FUNCTION_BLOCK FB_DirectControl EXTENDS FB_AsyncServiceResultClass IMPLEMENTS I_AcsiDataAccessEventClass, I_AcsiDataAccessCompletionClass
VAR
	(* Interface pointer to controllable DO *)
	_ipCtrl					: I_AcsiCommonControllableDataClass;
	(* CDC type of the controllable DO *)
	_eType					: E_AcsiCDCType;
	(* Interface pointer to value of 'Beh' DO of parent LN *)
	_ipBehVal				: I_AcsiDATypeBeh;
	(* Interface pointer to DO containing stepsize information for BAC *)
	_ipStepSize		: I_AcsiDATypeAnalogueValue;
	
	(* State of control state machine *)
	_eControlState			: E_DirectControlState;
	(* Interface pointer to association for the current control procedure *)
	_ipCurrentAA			: I_ScsmAssociationClass;
	(* IP address of the client for the current control procedure *)
	_stCurrrentIp			: ST_SockAddr;
	
	(* Interface pointer to LastApplError request service *)
	_ipLastApplErrorReq		: I_AsyncServiceResultClass;
	(* State of LastApplError transmission *)
	_nLastApplErrorReqState	: BYTE;
	(* Interface pointer to CommandTermination request service *)
	_ipCmdTermReq			: I_AsyncServiceResultClass;
	(* State of CommandTermination transmission *)
	_nCmdTermReqState		: BYTE;
	
	(* Indicates whether this function block has been initialized *)
	bInit					: BOOL;
	(* Indicates whether the ControlState changed in the last cycle *)
	bNewState				: BOOL;
	(* Indicates whether a valid Oper_req was received *)
	bOperReq				: BOOL;
	(* Token for CompletionWaitEvent *)
	fbCompletion			: FB_AcsiServiceResultClass;
END_VAR

(*
	Checks if the value of 'Oper.ctlVal' is valid.
	Return value: TRUE => success, FALSE => failure
*)
METHOD PROTECTED _CheckCtlVal : BOOL
VAR_INPUT
	(* Value of 'ctlVal' DA *)
	uCtlVal			: U_AcsiCtlVal;
END_VAR
VAR_OUTPUT
	(* Error *)
	eError			: E_AcsiApplError;
	(* Application error code *)
	eAddCause		: E_AcsiApplAddCause;
END_VAR
IF (_ipCtrl = 0) OR_ELSE (_eType = E_AcsiCDCType.none) THEN
	RETURN;
END_IF

CASE _eType OF
	E_AcsiCDCType.SPC:
		IF (_ipCtrl.ipStVal_BOOLEAN = 0) THEN
			RETURN;
		END_IF
		IF (uCtlVal.SPC = _ipCtrl.ipStVal_BOOLEAN.bValue) THEN
			eError:=E_AcsiApplError.NoError;
			eAddCause:=E_AcsiApplAddCause.PositionReached;
		ELSE
			_CheckCtlVal:=TRUE;
		END_IF
	
	E_AcsiCDCType.DPC:
		IF (_ipCtrl.ipStVal_Dbpos = 0) THEN
			RETURN;
		END_IF
		IF ((SEL(uCtlVal.DPC, E_AcsiDbpos.Off, E_AcsiDbpos.On)) = _ipCtrl.ipStVal_Dbpos.eValue) THEN
			eError:=E_AcsiApplError.NoError;
			eAddCause:=E_AcsiApplAddCause.PositionReached;
		ELSE
			_CheckCtlVal:=TRUE;
		END_IF
	
	E_AcsiCDCType.INC:
		IF (_ipCtrl.ipStVal_INT32 = 0) THEN
			RETURN;
		END_IF
		IF (uCtlVal.INC = _ipCtrl.ipStVal_INT32.iValue) THEN
			eError:=E_AcsiApplError.NoError;
			eAddCause:=E_AcsiApplAddCause.PositionReached;
		ELSE
			_CheckCtlVal:=TRUE;
		END_IF
		
	E_AcsiCDCType.ENC:
		IF (_ipCtrl.ipStVal_ENUMERATED = 0) THEN
			RETURN;
		END_IF
		IF (uCtlVal.ENC.iAny = _ipCtrl.ipStVal_ENUMERATED.iAny) THEN
			eError:=E_AcsiApplError.NoError;
			eAddCause:=E_AcsiApplAddCause.PositionReached;
		ELSE
			_CheckCtlVal:=TRUE;
		END_IF
	
	E_AcsiCDCType.BSC:
		IF (_ipCtrl.ipValWTr = 0) THEN
			RETURN;
		END_IF
		CASE uCtlVal.BSC OF
			E_AcsiTcmd.Reserved:
				eError:=E_AcsiApplError.NoError;
				eAddCause:=E_AcsiApplAddCause.NotSupported;
			
			E_AcsiTcmd.Lower:
				IF (_ipCtrl.ipValWTr.iPosVal = -64) THEN
					eError:=E_AcsiApplError.NoError;
					eAddCause:=E_AcsiApplAddCause.StepLimit;
				ELSE
					_CheckCtlVal:=TRUE;
				END_IF
			
			E_AcsiTcmd.Higher:
				IF (_ipCtrl.ipValWTr.iPosVal = 63) THEN
					eError:=E_AcsiApplError.NoError;
					eAddCause:=E_AcsiApplAddCause.StepLimit;
				ELSE
					_CheckCtlVal:=TRUE;
				END_IF
			
			E_AcsiTcmd.Stop:
				_CheckCtlVal:=TRUE;
		END_CASE
	
	E_AcsiCDCType.ISC:
		IF (_ipCtrl.ipValWTr = 0) THEN
			RETURN;
		END_IF
		IF (uCtlVal.ISC < -64) OR_ELSE (uCtlVal.ISC > 63) THEN
			eError:=E_AcsiApplError.NoError;
			eAddCause:=E_AcsiApplAddCause.InconsistentParameters;
		ELSE
			_CheckCtlVal:=TRUE;
		END_IF
	
	E_AcsiCDCType.APC:
		IF (_ipCtrl.ipMxVal = 0) THEN
			RETURN;
		ELSE
			_CheckCtlVal:=TRUE;
		END_IF
	
	E_AcsiCDCType.BAC:
		IF (_ipCtrl.ipMxVal = 0) THEN
			RETURN;
		ELSE
			CASE uCtlVal.BAC OF
				E_AcsiTcmd.Reserved:
					eError:=E_AcsiApplError.NoError;
					eAddCause:=E_AcsiApplAddCause.NotSupported;
				
				ELSE
					_CheckCtlVal:=TRUE;
			END_CASE
		END_IF
END_CASE
END_METHOD

(*
	This method performs the operative test.
	Since this test can take multiple PLC cycles, this method is called every cycle, until it returns TRUE.
*)
METHOD PROTECTED _DynamicTest : BOOL
VAR_OUTPUT
	(* Indicates whether the dynamic test was successful *)
	bDynamicTestOk	: BOOL;
	(* Error code for negative response *)
	eError			: E_AcsiServiceError;
END_VAR
bDynamicTestOk:=TRUE;
_DynamicTest:=TRUE;
END_METHOD

(* Initializes necessary local values *)
METHOD PROTECTED _Init
IF (_ipCtrl <> 0) THEN
	(* Set '_eType' according to CDC of the controllable data object *)
	IF (_ipCtrl.sClass = 'SPC') THEN
		_eType:=E_AcsiCDCType.SPC;
	ELSIF (_ipCtrl.sClass = 'DPC') THEN
		_eType:=E_AcsiCDCType.DPC;
	ELSIF (_ipCtrl.sClass = 'INC') THEN
		_eType:=E_AcsiCDCType.INC;
	ELSIF (_ipCtrl.sClass = 'ENC') THEN
		_eType:=E_AcsiCDCType.ENC;
	ELSIF (_ipCtrl.sClass = 'BSC') THEN
		_eType:=E_AcsiCDCType.BSC;
	ELSIF (_ipCtrl.sClass = 'ISC') THEN
		_eType:=E_AcsiCDCType.ISC;
	ELSIF (_ipCtrl.sClass = 'APC') THEN
		_eType:=E_AcsiCDCType.APC;
	ELSIF (_ipCtrl.sClass = 'BAC') THEN
		_eType:=E_AcsiCDCType.BAC;
	END_IF
END_IF
END_METHOD

(*
	This method performs the operative test.
	Since this test can take multiple PLC cycles, this method is called every cycle, until it returns TRUE.
*)
METHOD PROTECTED _OperativeTest : BOOL
VAR_OUTPUT
	(* Indicates whether the operative test was successful *)
	bOperativeTestOk	: BOOL;
	(* Error code for negative response *)
	eError				: E_AcsiServiceError;
END_VAR
VAR
	eApplError			: E_AcsiApplError;
	eApplAddCause		: E_AcsiApplAddCause;
END_VAR
IF (_ipCtrl <> 0) AND_THEN (_ipCtrl.ipOper <> 0) THEN
	(* Don't allow Oper_req if 'ctlModel' is set to 'status-only' *)
	IF (_ipCtrl.ipCtlModel <> 0) AND_THEN (_ipCtrl.ipCtlModel.eValue = E_AcsiCtlModels.StatusOnly) THEN
		_SendLastApplError(ipAA:=_ipCurrentAA,
			ipCtrlData:=_ipCtrl.ipOper,
			eError:=E_AcsiApplError.NoError,
			ipOrigin:=_ipCtrl.ipOper.ipOrigin,
			ipCtlNum:=_ipCtrl.ipOper.ipCtlNum,
			eAddCause:=E_AcsiApplAddCause.Unknown);
		eError:=E_AcsiServiceError.AccessViolation;
	
	(* Check if Oper_req is valid for current value of 'Beh' *)
	ELSIF (_ipBehVal <> 0) AND_THEN ((_ipBehVal.eValue = E_AcsiBeh.Off)
	OR_ELSE ((_ipCtrl.ipOper.ipTest <> 0) AND_THEN (_ipCtrl.ipOper.ipTest.bValue <> ((_ipBehVal.eValue = E_AcsiBeh.Test) OR_ELSE (_ipBehVal.eValue = E_AcsiBeh.TestBlocked))))) THEN
		_SendLastApplError(ipAA:=_ipCurrentAA,
			ipCtrlData:=_ipCtrl.ipOper,
			eError:=E_AcsiApplError.NoError,
			ipOrigin:=_ipCtrl.ipOper.ipOrigin,
			ipCtlNum:=_ipCtrl.ipOper.ipCtlNum,
			eAddCause:=E_AcsiApplAddCause.BlockedByMode);
		eError:=E_AcsiServiceError.AccessViolation;
	
	(* Check if 'ctlVal' is valid *)
	ELSIF (NOT _CheckCtlVal(uCtlVal:=_ipCtrl.ipOper.uCtlVal, eError=>eApplError, eAddCause=>eApplAddCause)) THEN
		_SendLastApplError(ipAA:=_ipCurrentAA,
			ipCtrlData:=_ipCtrl.ipOper,
			eError:=eApplError,
			ipOrigin:=_ipCtrl.ipOper.ipOrigin,
			ipCtlNum:=_ipCtrl.ipOper.ipCtlNum,
			eAddCause:=eApplAddCause);
		eError:=E_AcsiServiceError.AccessViolation;
	
	(* Oper_req is valid *)
	ELSE
		RemoteAddress_From_ScsmAssociation(in:=_ipCurrentAA, out=>_stCurrrentIp);
		bOperativeTestOk:=TRUE;
	END_IF
END_IF
_OperativeTest:=TRUE;
END_METHOD

(* Resets all local values and the ControlState *)
METHOD PROTECTED _Reset
(* Reset local values *)
_ipCurrentAA:=0;
_stCurrrentIp.sAddr:='';
_stCurrrentIp.nPort:=0;
END_METHOD

(* Resets all values of the 'Oper' DA to their configured initial values. *)
METHOD PROTECTED _ResetOperValues
VAR
	(* Interface pointer to 'Oper' DA *)
	ipOper			: I_AcsiDATypeOper;
END_VAR
IF (_ipCtrl = 0) OR_ELSE ((ipOper:=_ipCtrl.ipOper) = 0) THEN
	RETURN;
END_IF

IF (ipOper.ipCtlVal <> 0) THEN
	ipOper.uCtlVal:=ipOper.uCtlVal_Config;
END_IF
IF (ipOper.ipOperTm <> 0) THEN
	ipOper.ipOperTm.tValue:=ipOper.ipOperTm.tConfig;
END_IF
IF (ipOper.ipOrigin <> 0) THEN
	ipOper.ipOrigin.stOrigin:=ipOper.ipOrigin.stConfig;
END_IF
IF (ipOper.ipCtlNum <> 0) THEN
	ipOper.ipCtlNum.nValue:=ipOper.ipCtlNum.nConfig;
END_IF
IF (ipOper.ipT <> 0) THEN
	ipOper.ipT.tValue:=ipOper.ipT.tConfig;
END_IF
IF (ipOper.ipTest <> 0) THEN
	ipOper.ipTest.bValue:=ipOper.ipTest.bConfig;
END_IF
IF (ipOper.ipCheck <> 0) THEN
	ipOper.ipCheck.eValue:=ipOper.ipCheck.eConfig;
END_IF
END_METHOD

(* Sends a negative CommandTermination request *)
METHOD PROTECTED _SendCommandTerminationReqNeg : BOOL
VAR_INPUT
	(* Interface pointer to application association *)
	ipAA			: I_ScsmAssociationClass;
	(* Interface pointer to 'Oper', 'Cancel' or 'SBOw' control object, e.g. 'Relay1/XCBR1.CO.Pos.Oper', 'Relay1/CSWI1.CO.Pos.Cancel', 'Relay1/XCBR1.CO.Pos.SBOw' *)
	ipCtrlData		: I_AcsiCommonDataClass;
	(* Error *)
	eError			: E_AcsiApplError;
	(* Interface pointer to 'origin' attribute *)
	ipOrigin		: I_AcsiDATypeOriginator;
	(* Interface pointer to 'ctlNum' attribute *)
	ipCtlNum		: I_AcsiBAtypeINT8U;
	(* Application error code *)
	eAddCause		: E_AcsiApplAddCause;
END_VAR
VAR
	ipLastApplError	:I_AcsiDATypeLastApplError;
END_VAR
IF (ipAA <> 0)
AND_THEN (ipCtrlData <> 0)
AND_THEN (ipOrigin <> 0)
AND_THEN (ipCtlNum <> 0) THEN
	ipLastApplError:=ipAA.SetAdditionalCauseDiag(ipCtrlData:=ipCtrl,
		eError:=eError,
		stOrigin:=ipOrigin.stOrigin,
		nCtlNum:=ipCtlNum.nValue,
		eAddCause:=eAddCause);
	ipAA.CommandTerminationReq(ipCtrlData:=ipCtrlData,
		ipLastApplError:=ipLastApplError,
		ipResult=>_ipCmdTermReq);
	_nCmdTermReqState:=1;
END_IF
END_METHOD

(* Sends a positive CommandTermination request *)
METHOD PROTECTED _SendCommandTerminationReqPos : BOOL
VAR_INPUT
	(* Interface pointer to application association *)
	ipAA			: I_ScsmAssociationClass;
	(* Interface pointer to 'Oper', 'Cancel' or 'SBOw' control object, e.g. 'Relay1/XCBR1.CO.Pos.Oper', 'Relay1/CSWI1.CO.Pos.Cancel', 'Relay1/XCBR1.CO.Pos.SBOw' *)
	ipCtrlData		: I_AcsiCommonDataClass;
END_VAR
IF (ipAA <> 0)
AND_THEN (ipCtrlData <> 0) THEN
	_SendCommandTerminationReqPos:=ipAA.CommandTerminationReq(ipCtrlData:=ipCtrlData,
		ipLastApplError:=0,
		ipResult=>_ipCmdTermReq);
	_nCmdTermReqState:=1;
END_IF
END_METHOD

(* Sends a LastApplError request *)
METHOD PROTECTED _SendLastApplError : BOOL
VAR_INPUT
	(* Interface pointer to application association *)
	ipAA			: I_ScsmAssociationClass;
	(* Interface pointer to 'Oper', 'Cancel' or 'SBOw' control object *)
	ipCtrlData		: I_AcsiCommonDataClass;
	(* Error *)
	eError			: E_AcsiApplError;
	(* Interface pointer to 'origin' attribute *)
	ipOrigin		: I_AcsiDATypeOriginator;
	(* Interface pointer to 'ctlNum' attribute *)
	ipCtlNum		: I_AcsiBAtypeINT8U;
	(* Application error code *)
	eAddCause		: E_AcsiApplAddCause;
END_VAR
VAR
	(* Interface pointer to AdditionalCauseDiag object *)
	ipLastApplError	: I_AcsiDATypeLastApplError;
END_VAR
(* Get values from 'Oper' and send LastApplError *)
IF (ipAA <> 0) AND_THEN (ipOrigin <> 0) AND_THEN (ipCtlNum <> 0) THEN
	ipLastApplError:=ipAA.SetAdditionalCauseDiag(ipCtrlData:=ipCtrlData,
		eError:=eError,
		stOrigin:=ipOrigin.stOrigin,
		nCtlNum:=ipCtlNum.nValue,
		eAddCause:=eAddCause);
		
	_SendLastApplError:=ipAA.LastApplErrorReq(ipLastApplError:=ipLastApplError, ipResult=>_ipLastApplErrorReq);
	SUPER^.SetBusy();
	_nLastApplErrorReqState:=1;
END_IF
END_METHOD

(*
	Sets the value of 'mxVal' to the value of 'ctlVal'.
	Return value: TRUE => success, FALSE => failure
*)
METHOD PROTECTED _SetApcValue : BOOL
VAR_INPUT
	(* Interface pointer to DA that will be written *)
	ipMxVal			: I_AcsiDATypeAnalogueValue;
	(* Value of 'ctlVal' DA *)
	uCtlVal			: U_AcsiCtlVal;
	(* Interface pointer to 'ctlVal' of type AnalogueValue *)
	ipCtlVal_AV		: I_AcsiDATypeAnalogueValue;
END_VAR
VAR
END_VAR
IF ((ipMxVal = 0) OR_ELSE ((ipMxVal.ipF = 0) AND_THEN (ipMxVal.ipI = 0)))
OR_ELSE ((ipCtlVal_AV = 0) OR_ELSE ((ipCtlVal_AV.ipF = 0) AND_THEN (ipCtlVal_AV.ipI = 0))) THEN
	RETURN;
END_IF

IF (ipMxVal.ipF <> 0) THEN
	IF (ipCtlVal_AV.ipF <> 0) THEN
		ipMxVal.fValue:=uCtlVal.APC.f;
	ELSE
		(* 'ctlVal.i' is present, but not 'ctlVal.f' -> convert and use value of 'ctlVal.i' *)
		ipMxVal.fValue:=DINT_TO_REAL(uCtlVal.APC.i);
	END_IF
END_IF
IF (ipMxVal.ipI <> 0) THEN
	IF (ipCtlVal_AV.ipI <> 0) THEN
		ipMxVal.iValue:=uCtlVal.APC.i;
	ELSE
		(* 'ctlVal.f' is present, but not 'ctlVal.i' -> convert and use value of 'ctlVal.f' *)
		ipMxVal.iValue:=REAL_TO_DINT(uCtlVal.APC.f);
	END_IF
END_IF
_SetApcValue:=TRUE;
END_METHOD

(*
	Increments or decrements the value of 'mxVal' according to the value of 'ctlVal' and 'stepSize'.
	If 'stepSize' is not specified, the value 1 is used.
	Return value: TRUE => success, FALSE => failure
*)
METHOD PROTECTED _SetBacValue : BOOL
VAR_INPUT
	(* Interface pointer to DA that will be written *)
	ipMxVal			: I_AcsiDATypeAnalogueValue;
	(* Value of 'ctlVal' DA *)
	uCtlVal			: U_AcsiCtlVal;
	(* Interface pointer to 'stepSize' DA (Optional) *)
	ipStepSize		: I_AcsiDATypeAnalogueValue;
END_VAR
VAR
	(* stepSize for 'f' *)
	fStepSize		: REAL:=1.0;
	(* stepSize for 'i' *)
	iStepSize		: DINT:=1;
END_VAR
IF (ipMxVal = 0) OR_ELSE ((ipMxVal.ipF = 0) AND_THEN (ipMxVal.ipI = 0)) THEN
	RETURN;
END_IF

IF (ipStepSize <> 0) AND_THEN (((ipStepSize.ipF <> 0) AND_THEN (ipStepSize.fValue <> 0.0)) OR_ELSE ((ipStepSize.ipI <> 0) AND_THEN (ipStepSize.iValue <> 0))) THEN
	IF (ipStepSize.ipF <> 0) THEN
		fStepSize:=ipStepSize.fValue;
	ELSE
		(* 'stepSize.i' is present, but not 'stepSize.f' -> convert and use value of 'stepSize.i' *)
		fStepSize:=DINT_TO_REAL(ipStepSize.iValue);
	END_IF
	IF (ipStepSize.ipI <> 0) THEN
		iStepSize:=ipStepSize.iValue;
	ELSE
		(* 'stepSize.f' is present, but not 'stepSize.i' -> convert and use value of 'stepSize.f' *)
		iStepSize:=REAL_TO_DINT(ipStepSize.fValue);
	END_IF
END_IF

CASE uCtlVal.BAC OF
	E_AcsiTcmd.Stop:
		_SetBacValue:=TRUE;
	
	E_AcsiTcmd.Lower:
		IF (ipMxVal.ipF <> 0) THEN
			ipMxVal.fValue:=ipMxVal.fValue - fStepSize;
		END_IF
		IF (ipMxVal.ipI <> 0) THEN
			ipMxVal.iValue:=ipMxVal.iValue - iStepSize;
		END_IF
		_SetBacValue:=TRUE;
	
	E_AcsiTcmd.Higher:
		IF (ipMxVal.ipF <> 0) THEN
			ipMxVal.fValue:=ipMxVal.fValue + fStepSize;
		END_IF
		IF (ipMxVal.ipI <> 0) THEN
			ipMxVal.iValue:=ipMxVal.iValue + iStepSize;
		END_IF
		_SetBacValue:=TRUE;
END_CASE
END_METHOD

(*
	Increments or decrements the value of 'valWTr' according to the value of 'ctlVal'.
	Return value: TRUE => success, FALSE => failure
*)
METHOD PROTECTED _SetBscValue : BOOL
VAR_INPUT
	(* Interface pointer to DA that will be written *)
	ipValWTr		: I_AcsiDATypeValWithTrans;
	(* Value of 'ctlVal' DA *)
	uCtlVal			: U_AcsiCtlVal;
END_VAR
VAR
END_VAR
IF (ipValWTr = 0) THEN
	RETURN;
END_IF

CASE uCtlVal.BSC OF
	E_AcsiTcmd.Stop:
		_SetBscValue:=TRUE;
	
	E_AcsiTcmd.Lower:
		ipValWTr.iPosVal:=ipValWTr.iPosVal - 1;
		_SetBscValue:=TRUE;
	
	E_AcsiTcmd.Higher:
		ipValWTr.iPosVal:=ipValWTr.iPosVal + 1;
		_SetBscValue:=TRUE;
END_CASE
END_METHOD

(*
	Sets the value of 'stVal' according to the value of 'ctlVal'.
	Return value: TRUE => success, FALSE => failure
*)
METHOD PROTECTED _SetDpcValue : BOOL
VAR_INPUT
	(* Interface pointer to DA that will be written *)
	ipStVal			: I_AcsiDATypeDbpos;
	(* Value of 'ctlVal' DA *)
	uCtlVal			: U_AcsiCtlVal;
END_VAR
VAR
END_VAR
IF (ipStVal = 0) THEN
	RETURN;
END_IF

ipStVal.eValue:=SEL(uCtlVal.DPC, E_AcsiDbpos.Off, E_AcsiDbpos.On);
_SetDpcValue:=TRUE;
END_METHOD

(*
	Sets the value of 'stVal' to the value of 'ctlVal'.
	Return value: TRUE => success, FALSE => failure
*)
METHOD PROTECTED _SetEncValue : BOOL
VAR_INPUT
	(* Interface pointer to DA that will be written *)
	ipStVal			: I_AcsiBATypeENUMERATED;
	(* Value of 'ctlVal' DA *)
	uCtlVal			: U_AcsiCtlVal;
END_VAR
VAR
END_VAR
IF (ipStVal = 0) THEN
	RETURN;
END_IF

ipStVal.iAny:=uCtlVal.ENC.iAny;
_SetEncValue:=TRUE;
END_METHOD

(*
	Sets the value of 'stVal' to the value of 'ctlVal'.
	Return value: TRUE => success, FALSE => failure
*)
METHOD PROTECTED _SetIncValue : BOOL
VAR_INPUT
	(* Interface pointer to DA that will be written *)
	ipStVal			: I_AcsiBATypeINT32;
	(* Value of 'ctlVal' DA *)
	uCtlVal			: U_AcsiCtlVal;
END_VAR
VAR
END_VAR
IF (ipStVal = 0) THEN
	RETURN;
END_IF

ipStVal.iValue:=uCtlVal.INC;
_SetIncValue:=TRUE;
END_METHOD

(*
	Sets the value of 'valWTr' to the value of 'ctlVal'.
	Return value: TRUE => success, FALSE => failure
*)
METHOD PROTECTED _SetIscValue : BOOL
VAR_INPUT
	(* Interface pointer to DA that will be written *)
	ipValWTr		: I_AcsiDATypeValWithTrans;
	(* Value of 'ctlVal' DA *)
	uCtlVal			: U_AcsiCtlVal;
END_VAR
VAR
END_VAR
IF (ipValWTr = 0) THEN
	RETURN;
END_IF

ipValWTr.iPosVal:=uCtlVal.ISC;
_SetIscValue:=TRUE;
END_METHOD

(*
	Sets the value of 'stVal' to the value of 'ctlVal'.
	Return value: TRUE => success, FALSE => failure
*)
METHOD PROTECTED _SetSpcValue : BOOL
VAR_INPUT
	(* Interface pointer to DA that will be written *)
	ipStVal			: I_AcsiBATypeBOOLEAN;
	(* Value of 'ctlVal' DA *)
	uCtlVal			: U_AcsiCtlVal;
END_VAR
VAR
END_VAR
IF (ipStVal = 0) THEN
	RETURN;
END_IF

ipStVal.bValue:=uCtlVal.SPC;
_SetSpcValue:=TRUE;
END_METHOD

(*
	Sets the value of the respective DA according to the value of 'Oper.ctlVal'.
	Return value: TRUE => success, FALSE => failure
*)
METHOD PROTECTED _SetValue : BOOL
VAR_INPUT
	(* Value of 'ctlVal' DA *)
	uCtlVal			: U_AcsiCtlVal;
	(* Interface pointer to 'ctlVal' of type AnalogueValue *)
	ipCtlVal_AV		: I_AcsiDATypeAnalogueValue;
END_VAR
IF (_ipCtrl = 0) THEN
	RETURN;
END_IF

CASE _eType OF
	E_AcsiCDCType.SPC:
		_SetValue:=_SetSpcValue(ipStVal:=_ipCtrl.ipStVal_BOOLEAN, uCtlVal:=uCtlVal);
	
	E_AcsiCDCType.DPC:
		_SetValue:=_SetDpcValue(ipStVal:=_ipCtrl.ipStVal_Dbpos, uCtlVal:=uCtlVal);
	
	E_AcsiCDCType.INC:
		_SetValue:=_SetIncValue(ipStVal:=_ipCtrl.ipStVal_INT32, uCtlVal:=uCtlVal);
	
	E_AcsiCDCType.ENC:
		_SetValue:=_SetEncValue(ipStVal:=_ipCtrl.ipStVal_ENUMERATED, uCtlVal:=uCtlVal);
	
	E_AcsiCDCType.BSC:
		_SetValue:=_SetBscValue(ipValWTr:=_ipCtrl.ipValWTr, uCtlVal:=uCtlVal);
	
	E_AcsiCDCType.ISC:
		_SetValue:=_SetIscValue(ipValWTr:=_ipCtrl.ipValWTr, uCtlVal:=uCtlVal);
	
	E_AcsiCDCType.APC:
		_SetValue:=_SetApcValue(ipMxVal:=_ipCtrl.ipMxVal, uCtlVal:=uCtlVal, ipCtlVal_AV:=ipCtlVal_AV);
	
	E_AcsiCDCType.BAC:
		_SetValue:=_SetBacValue(ipMxVal:=_ipCtrl.ipMxVal, uCtlVal:=uCtlVal, ipStepSize:=_ipStepSize);
END_CASE
END_METHOD

(*
	Sets the value of 't' to the current time.
	Return value: TRUE => success, FALSE => failure
*)
METHOD PROTECTED _UpdateTimestampValue : BOOL
VAR_INPUT
	(* Interface pointer to association *)
	ipAA			: I_ScsmAssociationClass;
END_VAR
VAR
	(* Current time *)
	tValue			: T_UtcTime;
END_VAR
IF (ipAA <> 0) AND_THEN (_ipCtrl <> 0) AND_THEN (_ipCtrl.ipT <> 0) THEN
	_UpdateTimestampValue:=ipAA.GetSystemTime(tT=>tValue);
	_ipCtrl.ipT.tValue:=tValue;
END_IF
END_METHOD

PROPERTY eType : E_AcsiCDCType
GET
eType:=_eType;
END_GET
SET
_eType:=eType;
END_SET
END_PROPERTY

METHOD Execute : BOOL
VAR
	(* Used to cache the return value of the last '_OperativeTest' or '_DynamicTest' method call *)
	bTestOk	: BOOL;
	(* Used to cache the returned error of the last '_OperativeTest' or '_DynamicTest' method call *)
	eError	: E_AcsiServiceError;
	
	(* Used to cache the current system time for 'tOpOk' *)
	tValue	: T_UtcTime;
END_VAR
IF (_ipCtrl <> 0) AND_THEN (_ipCtrl.ipOper <> 0) THEN
	(* Initialize function block in the first cycle *)
	IF NOT bInit THEN
		_Init();
		bInit:=TRUE;
	END_IF
	
	CASE _eControlState OF
		E_DirectControlState.Ready:
			(* Check if ControlState changed in the last cycle *)
			IF bNewState THEN
				bNewState:=FALSE;
				_Reset();
			END_IF
			(* Check if a valid Oper_req was received *)
			IF bOperReq THEN
				bOperReq:=FALSE;
				(* Go to next ControlState *)
				_eControlState:=E_DirectControlState.PerformTest;
				bNewState:=TRUE;
			END_IF
		
		E_DirectControlState.PerformTest:
			(* Check if ControlState changed in the last cycle *)
			IF bNewState THEN
				bNewState:=FALSE;
				(* Set 'opRcvd' *)
				IF (_ipCtrl.ipOpRcvd <> 0) THEN
					_ipCtrl.ipOpRcvd.bValue:=TRUE;
				END_IF
			END_IF
			(* Trigger the operative test until it is finished *)
			IF _OperativeTest(bOperativeTestOk=>bTestOk, eError=>eError) THEN
				(* Reset 'opRcvd' *)
				IF (_ipCtrl.ipOpRcvd <> 0) THEN
					_ipCtrl.ipOpRcvd.bValue:=FALSE;
				END_IF
				IF bTestOk THEN
					(* Go to next ControlState *)
					_eControlState:=E_DirectControlState.WaitForExecution;
				ELSE
					fbCompletion.SetCompleted();
					fbCompletion.eServiceError:=eError;
					(* Go back to ControlState 'Ready' *)
					_eControlState:=E_DirectControlState.Ready;
				END_IF
				bNewState:=TRUE;
			END_IF
		
		E_DirectControlState.WaitForExecution:
			(* Check if ControlState changed in the last cycle *)
			IF bNewState THEN
				bNewState:=FALSE;
			END_IF
			(* Trigger the dynamic test until it is finished *)
			IF _DynamicTest(bDynamicTestOk=>bTestOk, eError=>eError) THEN
				fbCompletion.SetCompleted();
				IF bTestOk THEN
					(* Go to next ControlState *)
					IF (_ipBehVal <> 0) AND_THEN ((_ipBehVal.eValue = E_AcsiBeh.TestBlocked) OR_ELSE (_ipBehVal.eValue = E_AcsiBeh.OnBlocked)) THEN
						_eControlState:=E_DirectControlState.MirrorBlockedCommand;
					ELSE
						_eControlState:=E_DirectControlState.WaitForChange;
					END_IF
				ELSE
					fbCompletion.eServiceError:=eError;
					(* Go back to ControlState 'Ready' *)
					_eControlState:=E_DirectControlState.Ready;
				END_IF
				bNewState:=TRUE;
			END_IF
		
		E_DirectControlState.WaitForChange:
			(* Check if ControlState changed in the last cycle *)
			IF bNewState THEN
				bNewState:=FALSE;
				(* Set 'opOk' *)
				IF (_ipCtrl.ipOpOk <> 0) THEN
					_ipCtrl.ipOpOk.bValue:=TRUE;
				END_IF
				(* Set 'tOpOk' *)
				IF (_ipCtrl.ipTOpOk <> 0) AND_THEN (_ipCurrentAA <> 0) AND_THEN (_ipCurrentAA.GetSystemTime(tT=>tValue)) THEN
					_ipCtrl.ipTOpOk.tValue:=tValue;
				END_IF
			END_IF
			(* Update value *)
			_SetValue(uCtlVal:=_ipCtrl.ipOper.uCtlVal, ipCtlVal_AV:=_ipCtrl.ipOper.ipCtlVal_AnalogueValue);
			(* Update Timestamp 't' *)
			_UpdateTimestampValue(ipAA:=_ipCurrentAA);
			
			(* Reset 'opOk' *)
			IF (_ipCtrl.ipOpOk <> 0) THEN
				_ipCtrl.ipOpOk.bValue:=FALSE;
			END_IF
			(* Send CmdTerm_req+ *)
			_SendCommandTerminationReqPos(ipAA:=_ipCurrentAA, ipCtrlData:=_ipCtrl.ipOper);
			(* Go back to ControlState 'Ready' *)
			_eControlState:=E_DirectControlState.Ready;
			bNewState:=TRUE;
		
		E_DirectControlState.MirrorBlockedCommand:
			(* Check if ControlState changed in the last cycle *)
			IF bNewState THEN
				bNewState:=FALSE;
				(* Set 'opOk' *)
				IF (_ipCtrl.ipOpOk <> 0) THEN
					_ipCtrl.ipOpOk.bValue:=TRUE;
				END_IF
				(* Set 'tOpOk' *)
				IF (_ipCtrl.ipTOpOk <> 0) AND_THEN (_ipCurrentAA <> 0) AND_THEN (_ipCurrentAA.GetSystemTime(tT=>tValue)) THEN
					_ipCtrl.ipTOpOk.tValue:=tValue;
				END_IF
			END_IF
			(* Reset 'opOk' *)
			IF (_ipCtrl.ipOpOk <> 0) THEN
				_ipCtrl.ipOpOk.bValue:=FALSE;
			END_IF
			(* Send CmdTerm_req- *)
			_SendCommandTerminationReqNeg(ipAA:=_ipCurrentAA,
				ipCtrlData:=_ipCtrl.ipOper,
				eError:=E_AcsiApplError.NoError,
				ipOrigin:=_ipCtrl.ipOper.ipOrigin,
				ipCtlNum:=_ipCtrl.ipOper.ipCtlNum,
				eAddCause:=E_AcsiApplAddCause.BlockedByMode);
			(* Go back to ControlState 'Ready' *)
			_eControlState:=E_DirectControlState.Ready;
			bNewState:=TRUE;
	END_CASE
END_IF

(* Monitor transmission of LastApplError *)
CASE _nLastApplErrorReqState OF
	0:	;
	1:
		IF (_ipLastApplErrorReq <> 0) THEN
			Execute:=_ipLastApplErrorReq.Execute();
			IF NOT _ipLastApplErrorReq.IsBusy() THEN
				IF _ipLastApplErrorReq.IsCompleted() THEN
					SUPER^.SetCompleted();
				ELSE
					SUPER^.CopyFrom(ipSource:=_ipLastApplErrorReq);
				END_IF
				_nLastApplErrorReqState:=0;
			END_IF
		END_IF
END_CASE
(* Monitor transmission of CommandTermination *)
CASE _nCmdTermReqState OF
	0:	RETURN;
	1:
		IF (_ipCmdTermReq <> 0) THEN
			Execute:=_ipCmdTermReq.Execute();
			IF NOT _ipCmdTermReq.IsBusy() THEN
				IF _ipCmdTermReq.IsCompleted() THEN
					SUPER^.SetCompleted();
				ELSE
					SUPER^.CopyFrom(ipSource:=_ipLastApplErrorReq);
				END_IF
				_nCmdTermReqState:=0;
			END_IF
		END_IF
END_CASE
END_METHOD

PROPERTY ipBehVal : I_AcsiDATypeBeh
GET
ipBehVal:=_ipBehVal;
END_GET
SET
_ipBehVal:=ipBehVal;
END_SET
END_PROPERTY

PROPERTY ipCtrl : I_AcsiCommonControllableDataClass
GET
ipCtrl:=_ipCtrl;
END_GET
SET
IF (ipCtrl=0) THEN
	RETURN;
END_IF
_ipCtrl:=ipCtrl;
ipCtrl.ipEventSink:=THIS^;
END_SET
END_PROPERTY

PROPERTY ipStepSize : I_AcsiDATypeAnalogueValue
GET
ipStepSize:=_ipStepSize;
END_GET
SET
_ipStepSize:=ipStepSize;
END_SET
END_PROPERTY

METHOD OnAbort : BOOL
VAR_INPUT
	ipReason : I_ServiceErrorClass;
END_VAR
VAR_OUTPUT
	ipResult : I_AsyncServiceResultClass:=THIS^;
END_VAR
(* Forward Abort to LastApplError request service *)
IF (_ipLastApplErrorReq <> 0)AND_THEN (_ipLastApplErrorReq.IsBusy()) THEN
	_ipLastApplErrorReq.OnAbort(ipReason:=ipReason);
END_IF
(* Forward Abort to CommandTermination request service *)
IF (_ipCmdTermReq <> 0) AND_THEN (_ipCmdTermReq.IsBusy()) THEN
	_ipCmdTermReq.OnAbort(ipReason:=ipReason);
END_IF

SUPER^.SetCompleted();
fbCompletion.SetCompleted();
END_METHOD

METHOD OnCompletionWaitEvent : BOOL
VAR_INPUT
	ipDai			: I_AcsiDataAccessInfoClass;
	ipData			: I_AcsiCommonDataClass;
	eFc				: E_AcsiFc;
END_VAR
VAR_OUTPUT
	ipResult		: I_AcsiServiceResultClass;
END_VAR
VAR
	eServiceError	: E_AcsiServiceError;
END_VAR
fbCompletion.SetCompleted();
IF (ipDai = 0) OR_ELSE (ipData = 0) THEN
	fbCompletion.eServiceError:=E_AcsiServiceError.AccessViolation;
	RETURN;
END_IF

(* Check if an Operate request is received *)
(* Call the corresponing OnReq method and check if the control request is accepted *)
IF (ipDai.eService = E_AcsiServiceType.SetDataValues) AND_THEN (ipData.sObjectName = 'Oper') THEN
	ScsmAssociation_From_Dai(in:=ipDai, out=>_ipCurrentAA);
	fbCompletion.SetBusy();
	bOperReq:=TRUE;
	OnCompletionWaitEvent:=TRUE;
END_IF
END_METHOD

(* Implementation of user application data update event method. *)
METHOD OnGetVEvent
VAR_INPUT
	ipDai			: I_AcsiDataAccessInfoClass;(* Additional data access info *)
	ipData			: I_AcsiCommonDataClass;(* Interface pointer to data object *)
	eFc				: E_AcsiFc;(* Functional constraint *)
END_VAR
END_METHOD

(* Implementation of user application data update event method. *)
METHOD OnGetVPreEvent : E_AcsiServiceError
VAR_INPUT
	ipDai			: I_AcsiDataAccessInfoClass;(* Additional data access info *)
	ipData			: I_AcsiCommonDataClass;(* Interface pointer to data object *)
	eFc				: E_AcsiFc;(* Functional constraint *)
END_VAR
END_METHOD

(* Implementation of user application data update event method. *)
METHOD OnSetVEvent
VAR_INPUT
	ipDai			: I_AcsiDataAccessInfoClass;(* Additional data access info *)
	ipData			: I_AcsiCommonDataClass;(* Interface pointer to data object *)
	eFc				: E_AcsiFc;(* Functional constraint *)
END_VAR
END_METHOD

(* Implementation of user application data update event method. *)
METHOD OnSetVPreEvent : E_AcsiServiceError
VAR_INPUT
	ipDai			: I_AcsiDataAccessInfoClass;(* Additional data access info *)
	ipMemory		: I_AnyMemoryBuffer;(* Interface pointer to buffer containig new value data *)
	ipData			: I_AcsiCommonDataClass;(* Interface pointer to data object *)
	eFc				: E_AcsiFc;(* Functional constraint *)
END_VAR
VAR_OUTPUT
	ipLastApplError	: I_AcsiDATypeLastApplError;(* IF <> 0 => send LastApplError request *)
END_VAR
VAR
	(* Interface pointer to application association *)
	ipAA			: I_ScsmAssociationClass;
END_VAR
IF (eFc = E_AcsiFc.CO) AND_THEN (_ipCtrl <> 0) AND_THEN (ipDai <> 0) AND_THEN (ipDai.Write) AND_THEN (ipDai.ipAccessData <> 0)
AND_THEN ScsmAssociation_From_Dai(in:=ipDai, out=>ipAA) THEN
	IF (_ipCtrl.ipOper <> 0) AND_THEN (_ipCtrl.ipOper.ipOrigin <> 0) AND_THEN (_ipCtrl.ipOper.ipCtlNum <> 0) THEN
		(* Check for invalid write attemps to prevent 'Oper' from being overwritten while a control request is being executed *)
		IF (ipDai.ipAccessData.sObjectName = 'Oper') THEN
			(* Only allow 'Oper' requests in state 'Ready' *)
			IF (_eControlState <> E_DirectControlState.Ready) THEN
				ipLastApplError:=ipAA.SetAdditionalCauseDiag(ipCtrlData:=_ipCtrl.ipOper,
					eError:=E_AcsiApplError.NoError,
					stOrigin:=_ipCtrl.ipOper.ipOrigin.stOrigin,
					nCtlNum:=_ipCtrl.ipOper.ipCtlNum.nValue,
					eAddCause:=E_AcsiApplAddCause.CommandAlreadyInExecution);
				OnSetVPreEvent:=E_AcsiServiceError.AccessViolation;
			END_IF
		ELSE
			(* Don't allow write access to subdata of 'Oper' *)
			ipLastApplError:=ipAA.SetAdditionalCauseDiag(ipCtrlData:=_ipCtrl.ipOper,
				eError:=E_AcsiApplError.NoError,
				stOrigin:=_ipCtrl.ipOper.ipOrigin.stOrigin,
				nCtlNum:=_ipCtrl.ipOper.ipCtlNum.nValue,
				eAddCause:=E_AcsiApplAddCause.NotSupported);
			OnSetVPreEvent:=E_AcsiServiceError.AccessViolation;
		END_IF
	END_IF
END_IF
END_METHOD

END_FUNCTION_BLOCK
